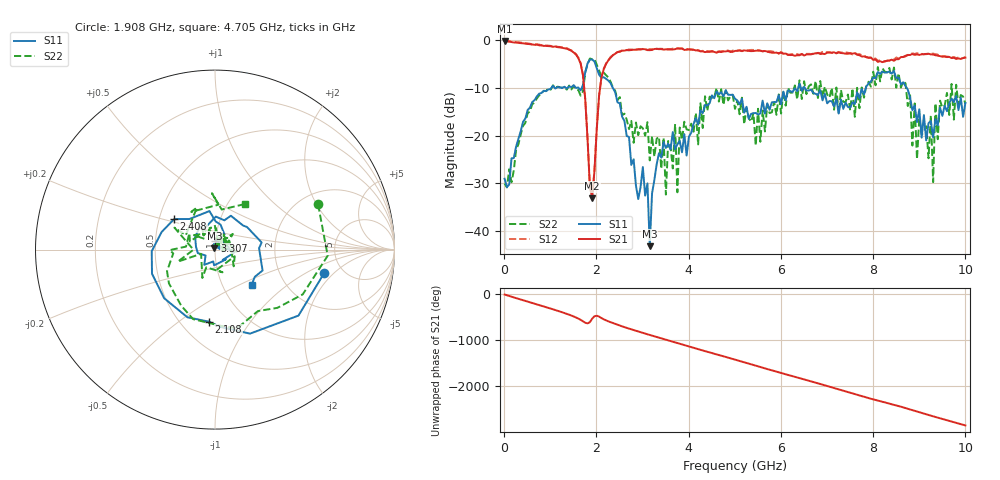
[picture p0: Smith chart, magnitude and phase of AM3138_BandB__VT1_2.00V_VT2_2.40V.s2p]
! Date/Time: Tue, Nov 13, 2018 4:39 PM
! Network Analyzer: Agilent Technologies E8364B Rev: A.07.50.67
! Sweep from 0.010 to 10.000 GHz, 201 Points, Sweep Type: LIN
! Power Supply: 2.001 V, 0.000 A
# Hz S DB R 50
!freq MagS11 AngS11 MagS21 AngS21 MagS12 AngS12 MagS22 AngS22
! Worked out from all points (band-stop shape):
!   201 points, 10 MHz to 10 GHz, reference 50 ohm
!   highest |S21| = -0.23 dB at 10 MHz (marker M1); lowest = -33.1 dB at 1.908 GHz (marker M2)
!   |S21| within 3 dB of the highest: start of sweep to 1.568 GHz; 2.357 GHz to 6.271 GHz (3.914 GHz wide, 90.7 % of centre)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
!   lowest |S11| = -43.1 dB at 3.157 GHz (marker M3), VSWR 1.01, Z = 49.7 + j0.626 ohm
!   |S11| at or under -10 dB: 2.353 GHz to 6.377 GHz (4.024 GHz wide, 92.2 % of centre); 6.516 GHz to 7.845 GHz (1.328 GHz wide, 18.5 % of centre); 8.725 GHz to end of sweep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
!   |S22| runs from -32.3 to -3.9 dB; largest |S21 - S12| = 0.037
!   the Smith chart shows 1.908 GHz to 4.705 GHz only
!   S11 on the Smith chart (normalised r, x): 1.908 GHz: 3.63, -1.52; 2.108 GHz: 0.68, -0.65; 2.408 GHz: 0.60, +0.22; 3.307 GHz: 0.99, +0.10; 4.705 GHz: 1.36, -0.59
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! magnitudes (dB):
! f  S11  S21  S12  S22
! 10 MHz  -29.0  -0.2  -0.1  -30.0
! 1.708 GHz  -9.5  -7.4  -7.3  -10.8
! 1.908 GHz  -4.1  -33.1  -33.1  -4.1
! 2.108 GHz  -7.9  -8.0  -7.8  -7.6
! 2.408 GHz  -10.9  -2.9  -2.9  -10.7
! 3.107 GHz  -30.0  -2.2  -2.1  -17.2
! 3.157 GHz  -43.1  -2.2  -2.0  -25.2
! 3.307 GHz  -26.0  -1.9  -1.9  -20.7
! 3.357 GHz  -23.7  -2.0  -1.9  -20.3
! 3.507 GHz  -22.6  -2.0  -1.9  -32.3
! 3.706 GHz  -22.9  -2.0  -1.8  -17.6
! 3.756 GHz  -21.8  -1.8  -1.8  -31.8
! 3.806 GHz  -21.1  -1.9  -1.8  -18.3
! 4.705 GHz  -10.9  -2.5  -2.4  -10.3
! 5.005 GHz  -12.3  -2.3  -2.1  -14.4
! 6.703 GHz  -11.1  -2.9  -2.9  -11.3
! 8.352 GHz  -6.6  -4.3  -4.3  -5.9
! 8.951 GHz  -17.2  -3.1  -2.8  -24.9
! 9.251 GHz  -17.0  -3.1  -2.9  -15.8
! 9.301 GHz  -20.4  -3.1  -2.9  -29.7
! 9.351 GHz  -16.6  -3.2  -3.0  -13.3
! 10 GHz  -13.2  -3.7  -3.6  -13.4
